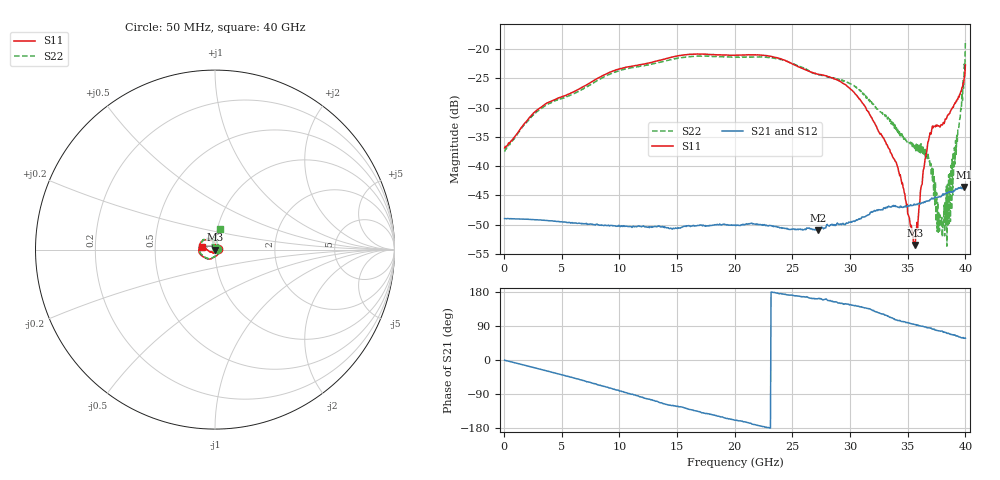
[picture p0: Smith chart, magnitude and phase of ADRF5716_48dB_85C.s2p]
! Device: ADRF5716
! Description: 30GHz 2-Bit Digital Attenuator
! Frequency: 100 MHz – 30 GHz
! Ports:
! ATTIN  = Port 1
! ATTOUT = Port 2
! State: 48 dB Attenuation selected
! Supply Voltage:
! VDD  =  +3.30 Volts
! VSS  =  -3.30 Volts
! Control Voltages:
! D5 = 3.3V, D6 = 3.3V
! Temperature = +85 C
! Data: Data was collected using a calibrated network analyzer.
!  The reference plane is the package pins of ADRF5716 switch.
! Note: Analog Devices supplies this data as a sample of measured data for this product.
!  Your particular data for this product may vary.
!  Analog Devices reserves the right to change this data at anytime
# HZ S DB R 50
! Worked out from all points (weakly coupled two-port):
!   800 points, 50 MHz to 40 GHz, reference 50 ohm
!   highest |S21| = -43.56 dB at 39.85 GHz (marker M1); lowest = -50.9 dB at 27.2 GHz (marker M2)
!   lowest |S11| = -53.5 dB at 35.65 GHz (marker M3), VSWR 1.00, Z = 50.2 - j0.0352 ohm
!   |S11| at or under -10 dB: start of sweep to end of sweep
!   |S22| runs from -53.7 to -18.5 dB; largest |S21 - S12| = 0
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5e7  -36.91 6.4  -48.97 -0.5  -48.97 -0.5  -37.52 4.7
2.8e9  -30.52 -53.1  -49.16 -21.8  -49.16 -21.8  -30.73 -52.6
6.75e9  -26.56 -103.4  -49.78 -53.2  -49.78 -53.2  -26.95 -104.2
9.65e9  -23.61 -127.3  -50.21 -78.4  -50.21 -78.4  -23.91 -128.5
1.34e10  -21.96 -152.7  -50.27 -111.2  -50.27 -111.2  -22.31 -155.5
2.005e10  -21.06 167.0  -50.07 -159.1  -50.07 -159.1  -21.37 161.4
2.4e10  -21.67 140.4  -50.53 175.4  -50.53 175.4  -21.74 134.1
2.67e10  -24.00 126.5  -50.75 162.8  -50.75 162.8  -24.06 114.3
2.72e10  -24.30 124.6  -50.93 161.5  -50.93 161.5  -24.37 112.1
3.035e10  -27.41 96.5  -49.38 143.5  -49.38 143.5  -26.26 83.1
3.335e10  -36.96 80.7  -46.85 114.4  -46.85 114.4  -32.09 51.9
3.42e10  -40.83 74.2  -47.02 104.0  -47.02 104.0  -33.76 42.3
3.545e10  -51.67 22.0  -46.72 95.0  -46.72 95.0  -36.12 23.8
3.565e10  -53.46 -9.5  -46.56 93.6  -46.56 93.6  -36.37 18.5
3.63e10  -41.75 -71.7  -46.23 88.6  -46.23 88.6  -38.01 -3.1
3.695e10  -34.31 -112.3  -45.70 84.8  -45.70 84.8  -40.14 -45.0
3.765e10  -33.09 -141.5  -45.32 77.1  -45.32 77.1  -51.29 -172.9
3.82e10  -32.47 -145.0  -44.77 73.4  -44.77 73.4  -51.93 -127.2
3.88e10  -30.27 -156.5  -44.38 67.2  -44.38 67.2  -47.51 145.0
3.965e10  -27.21 -178.3  -43.80 58.8  -43.80 58.8  -30.34 122.2
3.985e10  -25.75 172.6  -43.56 57.4  -43.56 57.4  -26.69 103.7
4e10  -22.73 168.3  -43.73 57.5  -43.73 57.5  -18.55 76.2
